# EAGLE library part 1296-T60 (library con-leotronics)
1.27mm SINGLE ROW FEMALE SOCKET Source: http://www.leotronics.co.uk/Conexcon/Data%20Sheets/sec.%20A/1296ing.pdf
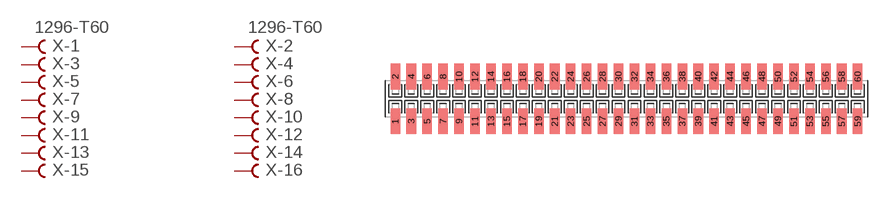
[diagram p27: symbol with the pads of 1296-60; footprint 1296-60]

Designator prefix X; gates -1=FVAL -2=FVAL -3=F -4=F -5=F -6=F -7=F -8=F -9=F -10=F -11=F -12=F -13=F -14=F -15=F -16=F -17=F -18=F -19=F -20=F -21=F -22=F -23=F -24=F -25=F -26=F -27=F -28=F -29=F -30=F -31=F -32=F -33=F -34=F -35=F -36=F -37=F -38=F -39=F -40=F -41=F -42=F -43=F -44=F -45=F -46=F -47=F -48=F -49=F -50=F -51=F -52=F -53=F -54=F -55=F -56=F -57=F -58=F -59=F -60=F

## 1296-T60 (OC_FARNELL: unknown; OC_NEWARK: unknown)  [1296-60]
1  -1:B  pas
2  -2:B  pas
3  -3:B  pas
4  -4:B  pas
5  -5:B  pas
6  -6:B  pas
7  -7:B  pas
8  -8:B  pas
9  -9:B  pas
10  -10:B  pas
11  -11:B  pas
12  -12:B  pas
13  -13:B  pas
14  -14:B  pas
15  -15:B  pas
16  -16:B  pas
17  -17:B  pas
18  -18:B  pas
19  -19:B  pas
20  -20:B  pas
21  -21:B  pas
22  -22:B  pas
23  -23:B  pas
24  -24:B  pas
25  -25:B  pas
26  -26:B  pas
27  -27:B  pas
28  -28:B  pas
29  -29:B  pas
30  -30:B  pas
31  -31:B  pas
32  -32:B  pas
33  -33:B  pas
34  -34:B  pas
35  -35:B  pas
36  -36:B  pas
37  -37:B  pas
38  -38:B  pas
39  -39:B  pas
40  -40:B  pas
41  -41:B  pas
42  -42:B  pas
43  -43:B  pas
44  -44:B  pas
45  -45:B  pas
46  -46:B  pas
47  -47:B  pas
48  -48:B  pas
49  -49:B  pas
50  -50:B  pas
51  -51:B  pas
52  -52:B  pas
53  -53:B  pas
54  -54:B  pas
55  -55:B  pas
56  -56:B  pas
57  -57:B  pas
58  -58:B  pas
59  -59:B  pas
60  -60:B  pas

## Footprint 1296-60 (pad centres in mm)
1.27mm SINGLE ROW FEMALE SOCKET Source: http://www.leotronics.co.uk/Conexcon/Data%20Sheets/sec.%20A/1296ing.pdf
smd 0.76 x 2.05: 1 -18.415,-1.78; 2 -18.415,1.78; 3 -17.145,-1.78; 4 -17.145,1.78; 5 -15.875,-1.78; 6 -15.875,1.78; 7 -14.605,-1.78; 8 -14.605,1.78; 9 -13.335,-1.78; 10 -13.335,1.78; 11 -12.065,-1.78; 12 -12.065,1.78; 13 -10.795,-1.78; 14 -10.795,1.78; 15 -9.525,-1.78; 16 -9.525,1.78; 17 -8.255,-1.78; 18 -8.255,1.78; 19 -6.985,-1.78; 20 -6.985,1.78; 21 -5.715,-1.78; 22 -5.715,1.78; 23 -4.445,-1.78; 24 -4.445,1.78; 25 -3.175,-1.78; 26 -3.175,1.78; 27 -1.905,-1.78; 28 -1.905,1.78; 29 -0.635,-1.78; 30 -0.635,1.78; 31 0.635,-1.78; 32 0.635,1.78; 33 1.905,-1.78; 34 1.905,1.78; 35 3.175,-1.78; 36 3.175,1.78; 37 4.445,-1.78; 38 4.445,1.78; 39 5.715,-1.78; 40 5.715,1.78; 41 6.985,-1.78; 42 6.985,1.78; 43 8.255,-1.78; 44 8.255,1.78; 45 9.525,-1.78; 46 9.525,1.78; 47 10.795,-1.78; 48 10.795,1.78; 49 12.065,-1.78; 50 12.065,1.78; 51 13.335,-1.78; 52 13.335,1.78; 53 14.605,-1.78; 54 14.605,1.78; 55 15.875,-1.78; 56 15.875,1.78; 57 17.145,-1.78; 58 17.145,1.78; 59 18.415,-1.78; 60 18.415,1.78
